(* Logix 5000 AddOnInstructionDefinition export EH_RA_5032_IOLink_8P_Promag10_Rev1; software revision 37.00 *)

TYPE EH_CommAOI_Data :
STRUCT
   Device_Comm_Error : BOOL;
   CommSuccess : BOOL;
   CommFailed : BOOL;
   CommTimeOut : BOOL;
   StateDone : BOOL;
   NewState : BOOL;
   OldState : SINT;
   PortSize : SINT;
   DevicePort : SINT;
   MaxState : SINT;
   State : SINT;
   VendorID : INT;
   DeviceID : DINT;
   CyclicData : INT[16];
   AcyclicData : DINT[8];
   ReplayIndex : INT;
   AOI_Diagnostic : DINT;
   ConnectionStatus : DINT;
   OutputData : INT[16];
END_STRUCT
END_TYPE

ADD_ON_INSTRUCTION EH_RA_5032_IOLink_8P_Promag10_Rev1   (* revision 1.1, vendor Endress+Hauser *)
// EH RA CommAOI 5032-8IOLxx 8P
// for the  Promag10 Rev.1
// Revision note:
// 1.1 Changed the Datatype from Unsigned to Signed
VAR_IN_OUT
   DataToSend : INT[10]; {required}
   CommAOIBusy : DINT; {required}
   ActiveComPort : DINT; {required}
   Send_Request : DINT; {required}
   CommError : INT; {required}
   DeviceData : EH_CommAOI_Data; {required}
   Device_Input : AB:5000_IOLINK_CC_2350E1D8:I:0; {required}
   Device_Output : AB:5000_IOLINK_CC_99E62D9B:O:0; {required}
   GetDeviceMSG : MESSAGE; {required}
   GetDeviceData : INT[10]; {required}
   SetDeviceMSG : MESSAGE; {required}
   SetDeviceData : INT[10]; {required}
END_VAR
VAR
   CopyDINT : DINT; {access None}
   StartValue : INT; {access None}
   UsedState : INT; {access None}
   cChannel : INT; {access None}
   DataSendExecuted : BOOL; {access None}
   MSG_Sent_Set : BOOL; {access None}
   MSG_Sent_Get : BOOL; {access None}
   ExecutionCounter : DINT; {access None}
   PortDint : DINT; {access None}
END_VAR

ROUTINE Logic   (* structured text *)
   // =======================================================================
   // Endress+Hauser Digital Solutions
   // ©Copyright (2024) All Rights Reserved
   // =======================================================================
   // Name:                EH_RA_5032_IOLink_CommAOI_8P_Promag10
   // Version:             1.1
   // Datum:               07.2025
   // Library:             01.00.01
   // Engineering:         Studio5000 V37.00.00
   // Author:              EH
   // =======================================================================
   
   if not Device_Input.ConnectionFaulted and Device_Input.RunMode then
   
   	//Device goes online if the correct device type is connected
   
   	DeviceData.DeviceID := 9728257;
   	DeviceData.VendorID := 17;
   	DeviceData.ConnectionStatus.0 := Device_Input.RunMode;
   
   	if Device_Input.ConnectionFaulted or Device_Input.Fault or Device_Input.DeviceError then
   
   		DeviceData.Device_Comm_Error := 1;
   
   	else
   
   		DeviceData.Device_Comm_Error := 0;
   
   	end_if;
   
   	PortDint := GetDeviceMSG.Path.DATA[GetDeviceMSG.Path.LEN-1];
   
   	case PortDint of
   
   		0:	DeviceData.DevicePort := 1;
   		2:	DeviceData.DevicePort := 2;
   		4:	DeviceData.DevicePort := 3;
   		6:	DeviceData.DevicePort := 4;
   		8:	DeviceData.DevicePort := 5;
   		10:	DeviceData.DevicePort := 6;
   		12:	DeviceData.DevicePort := 7;
   		14:	DeviceData.DevicePort := 8;
   
   		else
   
   			DeviceData.DevicePort := 0;
   
   	end_case;
   
   //Process Data Real to DINT
   // to use the Device AOI the Order has to be like the IODD
   
   	cop(Device_Input.ProcessDataIn.Volume_flow,CopyDINT,1);
   	StartValue := 0;  // In the DataArray for Process Data
   
   	DeviceData.CyclicData[StartValue+1].0	:= CopyDINT.0;
   	DeviceData.CyclicData[StartValue+1].1	:= CopyDINT.1;
   	DeviceData.CyclicData[StartValue+1].2	:= CopyDINT.2;
   	DeviceData.CyclicData[StartValue+1].3	:= CopyDINT.3;
   	DeviceData.CyclicData[StartValue+1].4	:= CopyDINT.4;
   	DeviceData.CyclicData[StartValue+1].5	:= CopyDINT.5;
   	DeviceData.CyclicData[StartValue+1].6	:= CopyDINT.6;
   	DeviceData.CyclicData[StartValue+1].7	:= CopyDINT.7;
   	DeviceData.CyclicData[StartValue+1].8	:= CopyDINT.8;
   	DeviceData.CyclicData[StartValue+1].9	:= CopyDINT.9;
   	DeviceData.CyclicData[StartValue+1].10	:= CopyDINT.10;
   	DeviceData.CyclicData[StartValue+1].11	:= CopyDINT.11;
   	DeviceData.CyclicData[StartValue+1].12	:= CopyDINT.12;
   	DeviceData.CyclicData[StartValue+1].13	:= CopyDINT.13;
   	DeviceData.CyclicData[StartValue+1].14	:= CopyDINT.14;
   	DeviceData.CyclicData[StartValue+1].15	:= CopyDINT.15;
   	DeviceData.CyclicData[StartValue].0	:= CopyDINT.16;
   	DeviceData.CyclicData[StartValue].1	:= CopyDINT.17;
   	DeviceData.CyclicData[StartValue].2	:= CopyDINT.18;
   	DeviceData.CyclicData[StartValue].3	:= CopyDINT.19;
   	DeviceData.CyclicData[StartValue].4	:= CopyDINT.20;
   	DeviceData.CyclicData[StartValue].5	:= CopyDINT.21;
   	DeviceData.CyclicData[StartValue].6	:= CopyDINT.22;
   	DeviceData.CyclicData[StartValue].7	:= CopyDINT.23;
   	DeviceData.CyclicData[StartValue].8	:= CopyDINT.24;
   	DeviceData.CyclicData[StartValue].9	:= CopyDINT.25;
   	DeviceData.CyclicData[StartValue].10	:= CopyDINT.26;
   	DeviceData.CyclicData[StartValue].11	:= CopyDINT.27;
   	DeviceData.CyclicData[StartValue].12	:= CopyDINT.28;
   	DeviceData.CyclicData[StartValue].13	:= CopyDINT.29;
   	DeviceData.CyclicData[StartValue].14	:= CopyDINT.30;
   	DeviceData.CyclicData[StartValue].15	:= CopyDINT.31;
   
   	cop(Device_Input.ProcessDataIn.Conductivity,CopyDINT,1);
   	StartValue := 2;
   
   	DeviceData.CyclicData[StartValue+1].0	:= CopyDINT.0;
   	DeviceData.CyclicData[StartValue+1].1	:= CopyDINT.1;
   	DeviceData.CyclicData[StartValue+1].2	:= CopyDINT.2;
   	DeviceData.CyclicData[StartValue+1].3	:= CopyDINT.3;
   	DeviceData.CyclicData[StartValue+1].4	:= CopyDINT.4;
   	DeviceData.CyclicData[StartValue+1].5	:= CopyDINT.5;
   	DeviceData.CyclicData[StartValue+1].6	:= CopyDINT.6;
   	DeviceData.CyclicData[StartValue+1].7	:= CopyDINT.7;
   	DeviceData.CyclicData[StartValue+1].8	:= CopyDINT.8;
   	DeviceData.CyclicData[StartValue+1].9	:= CopyDINT.9;
   	DeviceData.CyclicData[StartValue+1].10	:= CopyDINT.10;
   	DeviceData.CyclicData[StartValue+1].11	:= CopyDINT.11;
   	DeviceData.CyclicData[StartValue+1].12	:= CopyDINT.12;
   	DeviceData.CyclicData[StartValue+1].13	:= CopyDINT.13;
   	DeviceData.CyclicData[StartValue+1].14	:= CopyDINT.14;
   	DeviceData.CyclicData[StartValue+1].15	:= CopyDINT.15;
   	DeviceData.CyclicData[StartValue].0	:= CopyDINT.16;
   	DeviceData.CyclicData[StartValue].1	:= CopyDINT.17;
   	DeviceData.CyclicData[StartValue].2	:= CopyDINT.18;
   	DeviceData.CyclicData[StartValue].3	:= CopyDINT.19;
   	DeviceData.CyclicData[StartValue].4	:= CopyDINT.20;
   	DeviceData.CyclicData[StartValue].5	:= CopyDINT.21;
   	DeviceData.CyclicData[StartValue].6	:= CopyDINT.22;
   	DeviceData.CyclicData[StartValue].7	:= CopyDINT.23;
   	DeviceData.CyclicData[StartValue].8	:= CopyDINT.24;
   	DeviceData.CyclicData[StartValue].9	:= CopyDINT.25;
   	DeviceData.CyclicData[StartValue].10	:= CopyDINT.26;
   	DeviceData.CyclicData[StartValue].11	:= CopyDINT.27;
   	DeviceData.CyclicData[StartValue].12	:= CopyDINT.28;
   	DeviceData.CyclicData[StartValue].13	:= CopyDINT.29;
   	DeviceData.CyclicData[StartValue].14	:= CopyDINT.30;
   	DeviceData.CyclicData[StartValue].15	:= CopyDINT.31;
   
   	cop(Device_Input.ProcessDataIn.Temperature,CopyDINT,1);
   	StartValue := 4;
   
   	DeviceData.CyclicData[StartValue+1].0	:= CopyDINT.0;
   	DeviceData.CyclicData[StartValue+1].1	:= CopyDINT.1;
   	DeviceData.CyclicData[StartValue+1].2	:= CopyDINT.2;
   	DeviceData.CyclicData[StartValue+1].3	:= CopyDINT.3;
   	DeviceData.CyclicData[StartValue+1].4	:= CopyDINT.4;
   	DeviceData.CyclicData[StartValue+1].5	:= CopyDINT.5;
   	DeviceData.CyclicData[StartValue+1].6	:= CopyDINT.6;
   	DeviceData.CyclicData[StartValue+1].7	:= CopyDINT.7;
   	DeviceData.CyclicData[StartValue+1].8	:= CopyDINT.8;
   	DeviceData.CyclicData[StartValue+1].9	:= CopyDINT.9;
   	DeviceData.CyclicData[StartValue+1].10	:= CopyDINT.10;
   	DeviceData.CyclicData[StartValue+1].11	:= CopyDINT.11;
   	DeviceData.CyclicData[StartValue+1].12	:= CopyDINT.12;
   	DeviceData.CyclicData[StartValue+1].13	:= CopyDINT.13;
   	DeviceData.CyclicData[StartValue+1].14	:= CopyDINT.14;
   	DeviceData.CyclicData[StartValue+1].15	:= CopyDINT.15;
   	DeviceData.CyclicData[StartValue].0	:= CopyDINT.16;
   	DeviceData.CyclicData[StartValue].1	:= CopyDINT.17;
   	DeviceData.CyclicData[StartValue].2	:= CopyDINT.18;
   	DeviceData.CyclicData[StartValue].3	:= CopyDINT.19;
   	DeviceData.CyclicData[StartValue].4	:= CopyDINT.20;
   	DeviceData.CyclicData[StartValue].5	:= CopyDINT.21;
   	DeviceData.CyclicData[StartValue].6	:= CopyDINT.22;
   	DeviceData.CyclicData[StartValue].7	:= CopyDINT.23;
   	DeviceData.CyclicData[StartValue].8	:= CopyDINT.24;
   	DeviceData.CyclicData[StartValue].9	:= CopyDINT.25;
   	DeviceData.CyclicData[StartValue].10	:= CopyDINT.26;
   	DeviceData.CyclicData[StartValue].11	:= CopyDINT.27;
   	DeviceData.CyclicData[StartValue].12	:= CopyDINT.28;
   	DeviceData.CyclicData[StartValue].13	:= CopyDINT.29;
   	DeviceData.CyclicData[StartValue].14	:= CopyDINT.30;
   	DeviceData.CyclicData[StartValue].15	:= CopyDINT.31;
   
   	cop(Device_Input.ProcessDataIn.Totalizer_1_value,CopyDINT,1);
   	StartValue := 6;
   
   	DeviceData.CyclicData[StartValue+1].0	:= CopyDINT.0;
   	DeviceData.CyclicData[StartValue+1].1	:= CopyDINT.1;
   	DeviceData.CyclicData[StartValue+1].2	:= CopyDINT.2;
   	DeviceData.CyclicData[StartValue+1].3	:= CopyDINT.3;
   	DeviceData.CyclicData[StartValue+1].4	:= CopyDINT.4;
   	DeviceData.CyclicData[StartValue+1].5	:= CopyDINT.5;
   	DeviceData.CyclicData[StartValue+1].6	:= CopyDINT.6;
   	DeviceData.CyclicData[StartValue+1].7	:= CopyDINT.7;
   	DeviceData.CyclicData[StartValue+1].8	:= CopyDINT.8;
   	DeviceData.CyclicData[StartValue+1].9	:= CopyDINT.9;
   	DeviceData.CyclicData[StartValue+1].10	:= CopyDINT.10;
   	DeviceData.CyclicData[StartValue+1].11	:= CopyDINT.11;
   	DeviceData.CyclicData[StartValue+1].12	:= CopyDINT.12;
   	DeviceData.CyclicData[StartValue+1].13	:= CopyDINT.13;
   	DeviceData.CyclicData[StartValue+1].14	:= CopyDINT.14;
   	DeviceData.CyclicData[StartValue+1].15	:= CopyDINT.15;
   	DeviceData.CyclicData[StartValue].0	:= CopyDINT.16;
   	DeviceData.CyclicData[StartValue].1	:= CopyDINT.17;
   	DeviceData.CyclicData[StartValue].2	:= CopyDINT.18;
   	DeviceData.CyclicData[StartValue].3	:= CopyDINT.19;
   	DeviceData.CyclicData[StartValue].4	:= CopyDINT.20;
   	DeviceData.CyclicData[StartValue].5	:= CopyDINT.21;
   	DeviceData.CyclicData[StartValue].6	:= CopyDINT.22;
   	DeviceData.CyclicData[StartValue].7	:= CopyDINT.23;
   	DeviceData.CyclicData[StartValue].8	:= CopyDINT.24;
   	DeviceData.CyclicData[StartValue].9	:= CopyDINT.25;
   	DeviceData.CyclicData[StartValue].10	:= CopyDINT.26;
   	DeviceData.CyclicData[StartValue].11	:= CopyDINT.27;
   	DeviceData.CyclicData[StartValue].12	:= CopyDINT.28;
   	DeviceData.CyclicData[StartValue].13	:= CopyDINT.29;
   	DeviceData.CyclicData[StartValue].14	:= CopyDINT.30;
   	DeviceData.CyclicData[StartValue].15	:= CopyDINT.31;
   
   	// Temp value int to int
   	StartValue := 8;
   	DeviceData.CyclicData[StartValue].8	:= Device_Input.ProcessDataIn.Extended_device_status.0;
   	DeviceData.CyclicData[StartValue].9	:= Device_Input.ProcessDataIn.Extended_device_status.1;
   	DeviceData.CyclicData[StartValue].10	:= Device_Input.ProcessDataIn.Extended_device_status.2;
   	DeviceData.CyclicData[StartValue].11	:= Device_Input.ProcessDataIn.Extended_device_status.3;
   	DeviceData.CyclicData[StartValue].12	:= Device_Input.ProcessDataIn.Extended_device_status.4;
   	DeviceData.CyclicData[StartValue].13	:= Device_Input.ProcessDataIn.Extended_device_status.5;
   	DeviceData.CyclicData[StartValue].14	:= Device_Input.ProcessDataIn.Extended_device_status.6;
   	DeviceData.CyclicData[StartValue].15	:= Device_Input.ProcessDataIn.Extended_device_status.7;
   
   	// State IO Bit to Bit
   	StartValue := 8;
   
   	DeviceData.CyclicData[StartValue].0	:= Device_Input.ProcessDataIn.Switching_signal_channel_1_1_Vol_fl;
   	DeviceData.CyclicData[StartValue].1	:= Device_Input.ProcessDataIn.Switching_signal_channel_1_2_Vol_fl;
   	DeviceData.CyclicData[StartValue].2	:= Device_Input.ProcessDataIn.Switching_signal_channel_2_1_Conduct;
   	DeviceData.CyclicData[StartValue].3	:= Device_Input.ProcessDataIn.Switching_signal_channel_2_2_Conduct;
   	DeviceData.CyclicData[StartValue].4	:= Device_Input.ProcessDataIn.Switching_signal_channel_3_1_Temp;
   	DeviceData.CyclicData[StartValue].5	:= Device_Input.ProcessDataIn.Switching_signal_channel_3_2_Temp;
   	DeviceData.CyclicData[StartValue].6 := Device_Input.ProcessDataIn.Switching_signal_channel_4_1_Tot_1;
   	DeviceData.CyclicData[StartValue].7	:= Device_Input.ProcessDataIn.Switching_signal_channel_4_2_Tot_1;
   
   	//Output Definition
   
   	Device_Output.ProcessDataOut.Totalizer_1_Totalize := DeviceData.OutputData[0].9;
   	Device_Output.ProcessDataOut.Totalizer_1_Reset_hold := DeviceData.OutputData[0].8;
   	Device_Output.ProcessDataOut.Totalizer_1_Reset_totalize := DeviceData.OutputData[0].7;
   	Device_Output.ProcessDataOut.Totalizer_1_Hold := DeviceData.OutputData[0].6;
   	Device_Output.ProcessDataOut.Flow_override := DeviceData.OutputData[0].5;
   	Device_Output.ProcessDataOut.Device_search := DeviceData.OutputData[0].4;
   	Device_Output.ProcessDataOut.Control_signal_channel_4_Totalizer_1 := DeviceData.OutputData[0].3;
   	Device_Output.ProcessDataOut.Control_signal_channel_3_Temperature := DeviceData.OutputData[0].2;
   	Device_Output.ProcessDataOut.Control_signal_channel_2_Conductivity := DeviceData.OutputData[0].1;
   	Device_Output.ProcessDataOut.Control_signal_channel_1_Volume_flow := DeviceData.OutputData[0].0;
   
   else
   
   	DeviceData.ConnectionStatus := 0;
   
   end_if;
   
   
   if CommAOIBusy = 0 then
   
   	DeviceData.OldState := 0;
   	DeviceData.CommSuccess := 0;
   	DeviceData.CommTimeOut := 0;
   	DeviceData.ReplayIndex := 0;
   	DataSendExecuted := 0;
   	ExecutionCounter:= 0;
   	MSG_Sent_Get := 0;
   	MSG_Sent_Set := 0;
   
   end_if;
   
   	IF Send_Request > 0 and CommAOIBusy = 0 then
   
   		CommAOIBusy := 1;
   
   		for cChannel := 0 to 8 do
   
   			if Send_Request.[cChannel] then
   
   			ActiveComPort := cChannel;
   			// DataSendExecuted := 0;
   
   			exit;
   
   			end_if;
   
   		end_for;
   
   	end_if;
   
   // Read/Get ---- settings
   
   if CommAOIBusy = 1
   	and DeviceData.DevicePort = ActiveComPort
   	and DeviceData.State > 0
   	and DataToSend[5].7
   	and DeviceData.StateDone
   	and DataToSend[5].0
   	and DeviceData.State > DeviceData.OldState
   	and DeviceData.State < DeviceData.MaxState
   	and not DeviceData.CommSuccess
   	and not DeviceData.CommTimeOut
   	and not MSG_Sent_Get
   	and not DataSendExecuted then
   
   		GetDeviceMSG.Class := 267; // 0x10B
   		GetDeviceMSG.Instance:= DataToSend[3]; //IO-Link index number
   		GetDeviceMSG.Attribute := DataToSend[4];  //0 or Subindex nr (hex) not used
   		MSG_Sent_Get :=1;
   		DeviceData.ReplayIndex := GetDeviceMSG.Instance;
   		GetDeviceData[0] :=0;
   		GetDeviceData[1] :=0;
   		GetDeviceData[2] :=0;
   		GetDeviceData[3] :=0;
   		MSG(GetDeviceMSG);
   		DeviceData.NewState := 0;
   		DataSendExecuted := 1;
   
   end_if;
   
   // Write/Set -- settings
   
   if CommAOIBusy = 1
   	and DeviceData.DevicePort = ActiveComPort
   	and DeviceData.State > 0
   	and DataToSend[5].7
   	and DeviceData.StateDone
   	and DataToSend[5].1
   	and DeviceData.State > DeviceData.OldState
   	and DeviceData.State < DeviceData.MaxState
   	and not DataSendExecuted
   	and not DeviceData.CommSuccess
   	and not DeviceData.CommTimeOut
   	and not MSG_Sent_Set
   	and not DataSendExecuted then
   
   		SetDeviceMSG.Class := 267; // 0x10B
   		SetDeviceMSG.Instance:= DataToSend[3]; //IO-Link index number
   		SetDeviceMSG.Attribute := DataToSend[4];  //0 or Subindex nr (hex) not used
   		CopyDINT := 0;
   		CopyDINT.0 := DataToSend[5].8;
   		CopyDINT.1 := DataToSend[5].9;
   		CopyDINT.2 := DataToSend[5].10;
   		CopyDINT.3 := DataToSend[5].11;
   		CopyDINT.4 := DataToSend[5].12;
   		CopyDINT.5 := DataToSend[5].13;
   		CopyDINT.6 := DataToSend[5].14;
   		CopyDINT.7 := DataToSend[5].15;
   		SetDeviceMSG.REQ_LEN := CopyDINT;
   
   		SetDeviceData[0] := DataToSend[6];
   		SetDeviceData[1] := DataToSend[7];
   		SetDeviceData[2] := DataToSend[8];
   		SetDeviceData[3] := DataToSend[9];
   
   		DeviceData.ReplayIndex := SetDeviceMSG.Instance;
   		MSG_Sent_Set := 1;
   		MSG(SetDeviceMSG);
   		DeviceData.NewState := 0;
   		DataSendExecuted := 1;
   
   	end_if;
   
   	if SetDeviceMSG.DN
   		and DataSendExecuted
   		and DeviceData.State > DeviceData.OldState
   		and MSG_Sent_Set then
   
   		MSG_Sent_Set := 0;
   		DeviceData.CommSuccess := 1;
   		DeviceData.StateDone := 0;
   		DataSendExecuted := 0;
   
   	end_if;
   
   	if GetDeviceMSG.DN
   		and DataSendExecuted
   		and DeviceData.State > DeviceData.OldState
   		and MSG_Sent_Get then
   
   		case GetDeviceMSG.DN_LEN of
   
   			 1:
   
   				DeviceData.AcyclicData[0]	:= 0; // Reset Values
   				DeviceData.AcyclicData[1]	:= 0; // Reset Values
   				DeviceData.AcyclicData[0].0	:= GetDeviceData[0].0;
   				DeviceData.AcyclicData[0].1	:= GetDeviceData[0].1;
   				DeviceData.AcyclicData[0].2	:= GetDeviceData[0].2;
   				DeviceData.AcyclicData[0].3	:= GetDeviceData[0].3;
   				DeviceData.AcyclicData[0].4	:= GetDeviceData[0].4;
   				DeviceData.AcyclicData[0].5	:= GetDeviceData[0].5;
   				DeviceData.AcyclicData[0].6	:= GetDeviceData[0].6;
   				DeviceData.AcyclicData[0].7	:= GetDeviceData[0].7;
   
   				DeviceData.CommSuccess := 1;
   				MSG_Sent_Get := 0;
   				DeviceData.StateDone := 0;
   				DataSendExecuted := 0;
   
   			2:
   
   				DeviceData.AcyclicData[0]	:= 0; // Reset Values
   				DeviceData.AcyclicData[1]	:= 0; // Reset Values
   				DeviceData.AcyclicData[0].0	:= GetDeviceData[0].8;
   				DeviceData.AcyclicData[0].1	:= GetDeviceData[0].9;
   				DeviceData.AcyclicData[0].2	:= GetDeviceData[0].10;
   				DeviceData.AcyclicData[0].3	:= GetDeviceData[0].11;
   				DeviceData.AcyclicData[0].4	:= GetDeviceData[0].12;
   				DeviceData.AcyclicData[0].5	:= GetDeviceData[0].13;
   				DeviceData.AcyclicData[0].6	:= GetDeviceData[0].14;
   				DeviceData.AcyclicData[0].7	:= GetDeviceData[0].15;
   				DeviceData.AcyclicData[0].8	:= GetDeviceData[0].0;
   				DeviceData.AcyclicData[0].9	:= GetDeviceData[0].1;
   				DeviceData.AcyclicData[0].10	:= GetDeviceData[0].2;
   				DeviceData.AcyclicData[0].11	:= GetDeviceData[0].3;
   				DeviceData.AcyclicData[0].12	:= GetDeviceData[0].4;
   				DeviceData.AcyclicData[0].13	:= GetDeviceData[0].5;
   				DeviceData.AcyclicData[0].14	:= GetDeviceData[0].6;
   				DeviceData.AcyclicData[0].15	:= GetDeviceData[0].7;
   				DeviceData.CommSuccess := 1;
   				MSG_Sent_Get := 0;
   				DeviceData.StateDone := 0;
   				DataSendExecuted := 0;
   
   			4:
   
   				DeviceData.AcyclicData[0]	:= 0; // Reset Values
   				DeviceData.AcyclicData[1]	:= 0; // Reset Values
   				DeviceData.AcyclicData[0].0	:= GetDeviceData[1].8;
   				DeviceData.AcyclicData[0].1	:= GetDeviceData[1].9;
   				DeviceData.AcyclicData[0].2	:= GetDeviceData[1].10;
   				DeviceData.AcyclicData[0].3	:= GetDeviceData[1].11;
   				DeviceData.AcyclicData[0].4	:= GetDeviceData[1].12;
   				DeviceData.AcyclicData[0].5	:= GetDeviceData[1].13;
   				DeviceData.AcyclicData[0].6	:= GetDeviceData[1].14;
   				DeviceData.AcyclicData[0].7	:= GetDeviceData[1].15;
   				DeviceData.AcyclicData[0].8	:= GetDeviceData[1].0;
   				DeviceData.AcyclicData[0].9	:= GetDeviceData[1].1;
   				DeviceData.AcyclicData[0].10	:= GetDeviceData[1].2;
   				DeviceData.AcyclicData[0].11	:= GetDeviceData[1].3;
   				DeviceData.AcyclicData[0].12	:= GetDeviceData[1].4;
   				DeviceData.AcyclicData[0].13	:= GetDeviceData[1].5;
   				DeviceData.AcyclicData[0].14	:= GetDeviceData[1].6;
   				DeviceData.AcyclicData[0].15	:= GetDeviceData[1].7;
   				DeviceData.AcyclicData[0].16	:= GetDeviceData[0].8;
   				DeviceData.AcyclicData[0].17	:= GetDeviceData[0].9;
   				DeviceData.AcyclicData[0].18	:= GetDeviceData[0].10;
   				DeviceData.AcyclicData[0].19	:= GetDeviceData[0].11;
   				DeviceData.AcyclicData[0].20	:= GetDeviceData[0].12;
   				DeviceData.AcyclicData[0].21	:= GetDeviceData[0].13;
   				DeviceData.AcyclicData[0].22	:= GetDeviceData[0].14;
   				DeviceData.AcyclicData[0].23	:= GetDeviceData[0].15;
   				DeviceData.AcyclicData[0].24	:= GetDeviceData[0].0;;
   				DeviceData.AcyclicData[0].25	:= GetDeviceData[0].1;
   				DeviceData.AcyclicData[0].26	:= GetDeviceData[0].2;
   				DeviceData.AcyclicData[0].27	:= GetDeviceData[0].3;
   				DeviceData.AcyclicData[0].28	:= GetDeviceData[0].4;
   				DeviceData.AcyclicData[0].29	:= GetDeviceData[0].5;
   				DeviceData.AcyclicData[0].30	:= GetDeviceData[0].6;
   				DeviceData.AcyclicData[0].31	:= GetDeviceData[0].7;
   				DeviceData.CommSuccess := 1;
   				MSG_Sent_Get := 0;
   				DeviceData.StateDone := 0;
   				DataSendExecuted := 0;
   
   			6:
   
   				DeviceData.AcyclicData[0]	:= 0; // Reset Values
   				DeviceData.AcyclicData[1]	:= 0; // Reset Values
   				DeviceData.AcyclicData[0].0	:= GetDeviceData[1].8;
   				DeviceData.AcyclicData[0].1	:= GetDeviceData[1].9;
   				DeviceData.AcyclicData[0].2	:= GetDeviceData[1].10;
   				DeviceData.AcyclicData[0].3	:= GetDeviceData[1].11;
   				DeviceData.AcyclicData[0].4	:= GetDeviceData[1].12;
   				DeviceData.AcyclicData[0].5	:= GetDeviceData[1].13;
   				DeviceData.AcyclicData[0].6	:= GetDeviceData[1].14;
   				DeviceData.AcyclicData[0].7	:= GetDeviceData[1].15;
   				DeviceData.AcyclicData[0].8	:= GetDeviceData[1].0;
   				DeviceData.AcyclicData[0].9	:= GetDeviceData[1].1;
   				DeviceData.AcyclicData[0].10	:= GetDeviceData[1].2;
   				DeviceData.AcyclicData[0].11	:= GetDeviceData[1].3;
   				DeviceData.AcyclicData[0].12	:= GetDeviceData[1].4;
   				DeviceData.AcyclicData[0].13	:= GetDeviceData[1].5;
   				DeviceData.AcyclicData[0].14	:= GetDeviceData[1].6;
   				DeviceData.AcyclicData[0].15	:= GetDeviceData[1].7;
   				DeviceData.AcyclicData[0].16	:= GetDeviceData[0].8;
   				DeviceData.AcyclicData[0].17	:= GetDeviceData[0].9;
   				DeviceData.AcyclicData[0].18	:= GetDeviceData[0].10;
   				DeviceData.AcyclicData[0].19	:= GetDeviceData[0].11;
   				DeviceData.AcyclicData[0].20	:= GetDeviceData[0].12;
   				DeviceData.AcyclicData[0].21	:= GetDeviceData[0].13;
   				DeviceData.AcyclicData[0].22	:= GetDeviceData[0].14;
   				DeviceData.AcyclicData[0].23	:= GetDeviceData[0].15;
   				DeviceData.AcyclicData[0].24	:= GetDeviceData[0].0;;
   				DeviceData.AcyclicData[0].25	:= GetDeviceData[0].1;
   				DeviceData.AcyclicData[0].26	:= GetDeviceData[0].2;
   				DeviceData.AcyclicData[0].27	:= GetDeviceData[0].3;
   				DeviceData.AcyclicData[0].28	:= GetDeviceData[0].4;
   				DeviceData.AcyclicData[0].29	:= GetDeviceData[0].5;
   				DeviceData.AcyclicData[0].30	:= GetDeviceData[0].6;
   				DeviceData.AcyclicData[0].31	:= GetDeviceData[0].7;
   
   				DeviceData.AcyclicData[1].0	:= GetDeviceData[2].8;
   				DeviceData.AcyclicData[1].1	:= GetDeviceData[2].9;
   				DeviceData.AcyclicData[1].2	:= GetDeviceData[2].10;
   				DeviceData.AcyclicData[1].3	:= GetDeviceData[2].11;
   				DeviceData.AcyclicData[1].4	:= GetDeviceData[2].12;
   				DeviceData.AcyclicData[1].5	:= GetDeviceData[2].13;
   				DeviceData.AcyclicData[1].6	:= GetDeviceData[2].14;
   				DeviceData.AcyclicData[1].7	:= GetDeviceData[2].15;
   				DeviceData.AcyclicData[1].8	:= GetDeviceData[2].0;
   				DeviceData.AcyclicData[1].9	:= GetDeviceData[2].1;
   				DeviceData.AcyclicData[1].10	:= GetDeviceData[2].2;
   				DeviceData.AcyclicData[1].11	:= GetDeviceData[2].3;
   				DeviceData.AcyclicData[1].12	:= GetDeviceData[2].4;
   				DeviceData.AcyclicData[1].13	:= GetDeviceData[2].5;
   				DeviceData.AcyclicData[1].14	:= GetDeviceData[2].6;
   				DeviceData.AcyclicData[1].15	:= GetDeviceData[2].7;
   
   				DeviceData.CommSuccess := 1;
   				MSG_Sent_Get := 0;
   				DeviceData.StateDone := 0;
   				DataSendExecuted := 0;
   
   			8:
   
   				DeviceData.AcyclicData[0]	:= 0; // Reset Values
   				DeviceData.AcyclicData[1]	:= 0; // Reset Values
   				DeviceData.AcyclicData[0].0	:= GetDeviceData[1].8;
   				DeviceData.AcyclicData[0].1	:= GetDeviceData[1].9;
   				DeviceData.AcyclicData[0].2	:= GetDeviceData[1].10;
   				DeviceData.AcyclicData[0].3	:= GetDeviceData[1].11;
   				DeviceData.AcyclicData[0].4	:= GetDeviceData[1].12;
   				DeviceData.AcyclicData[0].5	:= GetDeviceData[1].13;
   				DeviceData.AcyclicData[0].6	:= GetDeviceData[1].14;
   				DeviceData.AcyclicData[0].7	:= GetDeviceData[1].15;
   				DeviceData.AcyclicData[0].8	:= GetDeviceData[1].0;
   				DeviceData.AcyclicData[0].9	:= GetDeviceData[1].1;
   				DeviceData.AcyclicData[0].10	:= GetDeviceData[1].2;
   				DeviceData.AcyclicData[0].11	:= GetDeviceData[1].3;
   				DeviceData.AcyclicData[0].12	:= GetDeviceData[1].4;
   				DeviceData.AcyclicData[0].13	:= GetDeviceData[1].5;
   				DeviceData.AcyclicData[0].14	:= GetDeviceData[1].6;
   				DeviceData.AcyclicData[0].15	:= GetDeviceData[1].7;
   				DeviceData.AcyclicData[0].16	:= GetDeviceData[0].8;
   				DeviceData.AcyclicData[0].17	:= GetDeviceData[0].9;
   				DeviceData.AcyclicData[0].18	:= GetDeviceData[0].10;
   				DeviceData.AcyclicData[0].19	:= GetDeviceData[0].11;
   				DeviceData.AcyclicData[0].20	:= GetDeviceData[0].12;
   				DeviceData.AcyclicData[0].21	:= GetDeviceData[0].13;
   				DeviceData.AcyclicData[0].22	:= GetDeviceData[0].14;
   				DeviceData.AcyclicData[0].23	:= GetDeviceData[0].15;
   				DeviceData.AcyclicData[0].24	:= GetDeviceData[0].0;;
   				DeviceData.AcyclicData[0].25	:= GetDeviceData[0].1;
   				DeviceData.AcyclicData[0].26	:= GetDeviceData[0].2;
   				DeviceData.AcyclicData[0].27	:= GetDeviceData[0].3;
   				DeviceData.AcyclicData[0].28	:= GetDeviceData[0].4;
   				DeviceData.AcyclicData[0].29	:= GetDeviceData[0].5;
   				DeviceData.AcyclicData[0].30	:= GetDeviceData[0].6;
   				DeviceData.AcyclicData[0].31	:= GetDeviceData[0].7;
   
   				DeviceData.AcyclicData[1].0	:= GetDeviceData[3].8;
   				DeviceData.AcyclicData[1].1	:= GetDeviceData[3].9;
   				DeviceData.AcyclicData[1].2	:= GetDeviceData[3].10;
   				DeviceData.AcyclicData[1].3	:= GetDeviceData[3].11;
   				DeviceData.AcyclicData[1].4	:= GetDeviceData[3].12;
   				DeviceData.AcyclicData[1].5	:= GetDeviceData[3].13;
   				DeviceData.AcyclicData[1].6	:= GetDeviceData[3].14;
   				DeviceData.AcyclicData[1].7	:= GetDeviceData[3].15;
   				DeviceData.AcyclicData[1].8	:= GetDeviceData[3].0;
   				DeviceData.AcyclicData[1].9	:= GetDeviceData[3].1;
   				DeviceData.AcyclicData[1].10	:= GetDeviceData[3].2;
   				DeviceData.AcyclicData[1].11	:= GetDeviceData[3].3;
   				DeviceData.AcyclicData[1].12	:= GetDeviceData[3].4;
   				DeviceData.AcyclicData[1].13	:= GetDeviceData[3].5;
   				DeviceData.AcyclicData[1].14	:= GetDeviceData[3].6;
   				DeviceData.AcyclicData[1].15	:= GetDeviceData[3].7;
   				DeviceData.AcyclicData[1].16	:= GetDeviceData[2].8;
   				DeviceData.AcyclicData[1].17	:= GetDeviceData[2].9;
   				DeviceData.AcyclicData[1].18	:= GetDeviceData[2].10;
   				DeviceData.AcyclicData[1].19	:= GetDeviceData[2].11;
   				DeviceData.AcyclicData[1].20	:= GetDeviceData[2].12;
   				DeviceData.AcyclicData[1].21	:= GetDeviceData[2].13;
   				DeviceData.AcyclicData[1].22	:= GetDeviceData[2].14;
   				DeviceData.AcyclicData[1].23	:= GetDeviceData[2].15;
   				DeviceData.AcyclicData[1].24	:= GetDeviceData[2].0;;
   				DeviceData.AcyclicData[1].25	:= GetDeviceData[2].1;
   				DeviceData.AcyclicData[1].26	:= GetDeviceData[2].2;
   				DeviceData.AcyclicData[1].27	:= GetDeviceData[2].3;
   				DeviceData.AcyclicData[1].28	:= GetDeviceData[2].4;
   				DeviceData.AcyclicData[1].29	:= GetDeviceData[2].5;
   				DeviceData.AcyclicData[1].30	:= GetDeviceData[2].6;
   				DeviceData.AcyclicData[1].31	:= GetDeviceData[2].7;
   
   				DeviceData.CommSuccess := 1;
   				MSG_Sent_Get := 0;
   				DeviceData.StateDone := 0;
   				DataSendExecuted := 0;
   
   		end_case;
   
   	end_if;
   
   	if SetDeviceMSG.ER and MSG_Sent_Set then
   
   		DeviceData.AOI_Diagnostic.[DeviceData.State+7] := 1;
   		DeviceData.CommTimeOut := 1;
   		MSG_Sent_Set := 0;
   		DeviceData.StateDone := 0;
   		DataSendExecuted := 0;
   
   	end_if;
   
   	if GetDeviceMSG.ER  and MSG_Sent_Get then
   
   		DeviceData.AOI_Diagnostic.[DeviceData.State+7] := 1;
   		DeviceData.CommTimeOut := 1;
   		MSG_Sent_Get := 0;
   		DeviceData.StateDone := 0;
   		DataSendExecuted := 0;
   
   	end_if;
   
   
   
END_ROUTINE
END_ADD_ON_INSTRUCTION
